(* Logix 5000 AddOnInstructionDefinition export B256_DINTtoE; software revision 30.00 *)

ADD_ON_INSTRUCTION D_SHR   (* revision 1.0, vendor Ken Fischer, NSWCPD, C512 *)
// DINT bit shift right of the 32-bit argument Inp_A by Inp_B bits with paddding by zeros on the right
// Revision note:
// Rev1.0: TBD - Initial Release
VAR_IN_OUT
   Inp_A : DINT; {required}   // 64-bit Integer to be right circular rotated
END_VAR
VAR_INPUT
   Inp_B : INT; {required}   // Number of bits to shift
END_VAR
VAR_IN_OUT
   Out : DINT; {required}   // Result
END_VAR
VAR
   BSR_Cntrl : CONTROL := (LEN := 32);
   ONS : BOOL;
   Source_Bit : BOOL;
   Wrk_InpA : DINT[2];
END_VAR

ROUTINE Logic   (* ladder *)
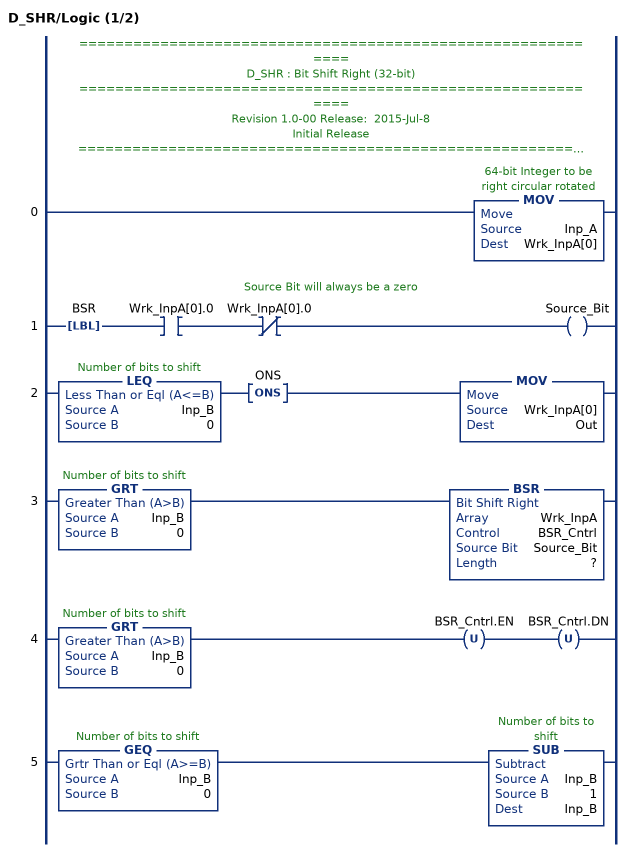
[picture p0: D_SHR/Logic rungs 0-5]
   // ============================================================
   // D_SHR : Bit Shift Right (32-bit)
   // ============================================================
   // Revision 1.0-00 Release:  2015-Jul-8
   // Initial Release
   // ============================================================
   // Performs a right bit shift of the 32-bit argument Inp_A by the
   // number of bits defined in the 16-bit argument Inp_B, with padding by zeros.
   0: MOV(Inp_A,Wrk_InpA[0]);
   // Source Bit will always be a zero
   1: LBL(BSR)XIC(Wrk_InpA[0].0)XIO(Wrk_InpA[0].0)OTE(Source_Bit);
   2: LEQ(Inp_B,0)ONS(ONS)MOV(Wrk_InpA[0],Out);
   3: GRT(Inp_B,0)BSR(Wrk_InpA,BSR_Cntrl,Source_Bit,?);
   4: GRT(Inp_B,0)OTU(BSR_Cntrl.EN)OTU(BSR_Cntrl.DN);
   5: GEQ(Inp_B,0)SUB(Inp_B,1,Inp_B);
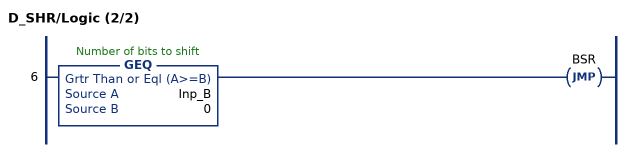
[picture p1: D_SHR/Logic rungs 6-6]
   6: GEQ(Inp_B,0)JMP(BSR);
END_ROUTINE
END_ADD_ON_INSTRUCTION

ADD_ON_INSTRUCTION B256_DINTtoE   (* revision 1.0 20170916, vendor Kenneth A. Fischer *)
// Convert 256-bit value using 8 32-bit pieces into 256-bit value using 32 8-bit pieces
// Revision note:
// Rev1.0: 20170916 - Initial Release
VAR_IN_OUT
   Inp_DINT : DINT[8]; {required}
   Out_E : DINT[32]; {required}
END_VAR
VAR
   i : INT;
   j : INT;
   D_SHR : D_SHR;
   TEMP : DINT;
END_VAR

ROUTINE Logic   (* ladder *)
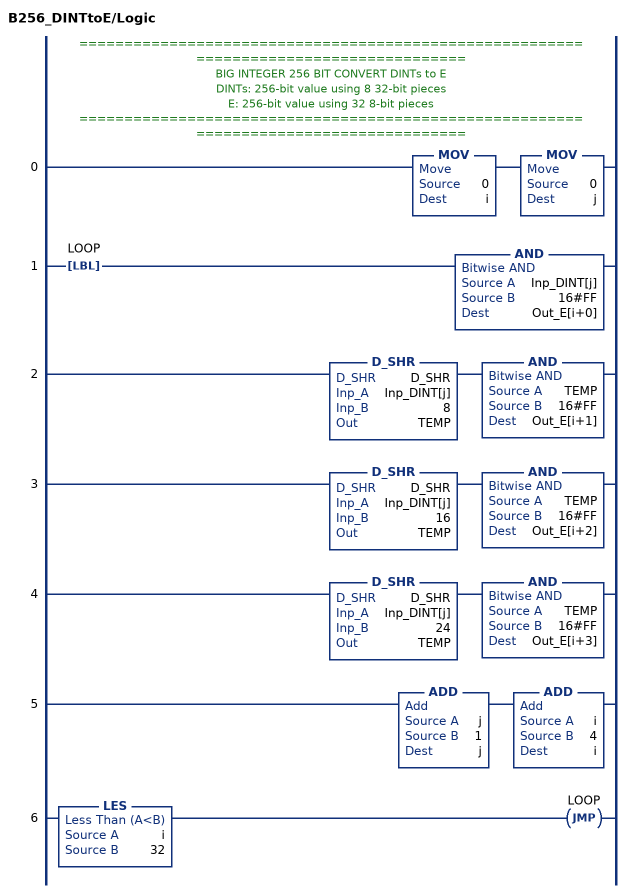
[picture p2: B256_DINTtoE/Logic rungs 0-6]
   // ======================================================================================
   // BIG INTEGER 256 BIT CONVERT DINTs to E
   // DINTs: 256-bit value using 8 32-bit pieces
   // E: 256-bit value using 32 8-bit pieces
   // ======================================================================================
   0: MOV(0,i)MOV(0,j);
   1: LBL(LOOP)AND(Inp_DINT[j],16#FF,Out_E[i+0]);
   2: D_SHR(D_SHR,Inp_DINT[j],8,TEMP)AND(TEMP,16#FF,Out_E[i+1]);
   3: D_SHR(D_SHR,Inp_DINT[j],16,TEMP)AND(TEMP,16#FF,Out_E[i+2]);
   4: D_SHR(D_SHR,Inp_DINT[j],24,TEMP)AND(TEMP,16#FF,Out_E[i+3]);
   5: ADD(j,1,j)ADD(i,4,i);
   6: LES(i,32)JMP(LOOP);
END_ROUTINE
END_ADD_ON_INSTRUCTION
